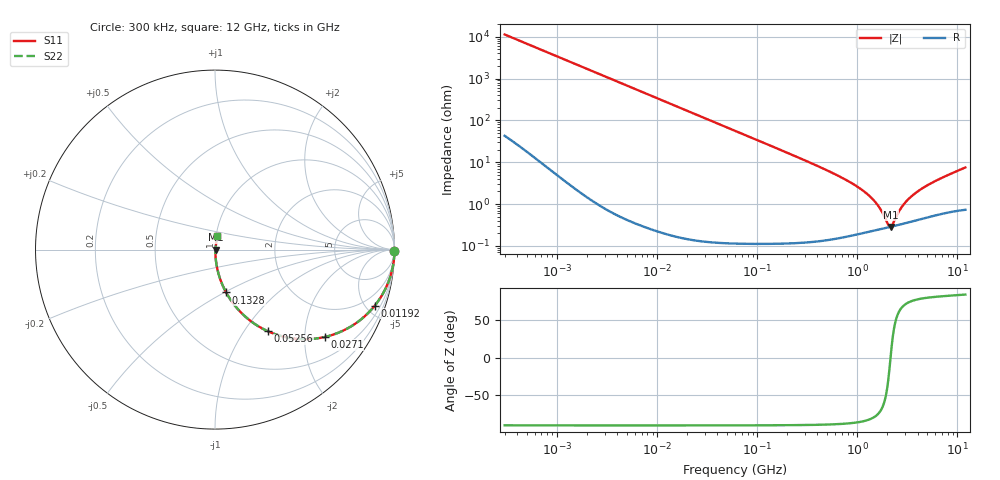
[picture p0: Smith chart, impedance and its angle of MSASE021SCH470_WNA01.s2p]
! MSASE021SCH470_WNA01  S-PARAMETER MODEL  ( Standard Model )
! Model Generated by TAIYO YUDEN Corporation (http://www.ty-top.com)
! Version 3.0
! TAIYO YUDEN Control No. 231201
! Copyright(c) 2016 TAIYO YUDEN CO.,LTD. All Rights Reserved.
! Product Description (link to TY-COMPAS)
! https://ds.yuden.co.jp/TYCOMPAS/or/detail?pn=MSASE021SCH470JWNA01&u=M
! Products Name : Multilayer Ceramic Capacitors
! Characteristics :
!  Capacitance : 47 [pF] , Rated Voltage : 16 [V] , TCC : CH / C0H
!  Case Size : 0.25 x 0.125 / 0.0098 x 0.0049 [mm/inch] , Thickness : 0.125 / 0.0049 [mm/inch]
!  (Conditions: Temperature = 25 [degC] , DC Bias Voltage = 0 [V])
! External Node Assignments :
!  1  o---| |---o  2
! GND o---------o GND
! Frequency Range : 0.3MHz  -  12000MHz  [ 401 STEP ]
# MHZ S RI R 50
! Freq[MHz].  S11 Real  S11 Imag  S21 Real  S21 Imag  S12 Real  S12 Imag  S22 Real  S22 Imag
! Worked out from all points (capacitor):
!   401 points, 300 kHz to 12 GHz, reference 50 ohm
!   read as one part in series: C = 47 pF near 316.3 kHz
!   lowest |Z| = 286 mohm at 2.145 GHz (marker M1)
!   series resonance near 2.145 GHz, so ESL is about 120 pH
!   S11 on the Smith chart (normalised r, x): 300 kHz: open; 11.92 MHz: 1.00, -5.69; 27.1 MHz: 1.00, -2.50; 52.56 MHz: 1.00, -1.29; 132.8 MHz: 1.00, -0.51; 12 GHz: 1.01, +0.15
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0.3  0.9999 -0.00886  0.000112 0.00886  0.000112 0.00886  0.9999 -0.00886
1.769972  0.9972 -0.052  0.00276 0.052  0.00276 0.052  0.9972 -0.052
4.593584  0.9819 -0.1329  0.0181 0.1329  0.0181 0.1329  0.9819 -0.1329
10.44266  0.9133 -0.281  0.0867 0.281  0.0867 0.281  0.9133 -0.281
11.92167  0.89 -0.3126  0.11 0.3126  0.11 0.3126  0.89 -0.3126
17.7384  0.7852 -0.4103  0.2148 0.4103  0.2148 0.4103  0.7852 -0.4103
27.10171  0.6104 -0.4871  0.3896 0.4871  0.3896 0.4871  0.6104 -0.4871
52.55639  0.2943 -0.4549  0.7057 0.4549  0.7057 0.4549  0.2943 -0.4549
60  0.2425 -0.4276  0.7575 0.4276  0.7575 0.4276  0.2425 -0.4276
86.94074  0.1325 -0.3376  0.8675 0.3376  0.8675 0.3376  0.1325 -0.3376
132.8329  0.0617 -0.2384  0.9383 0.2384  0.9383 0.2384  0.0617 -0.2384
353.9943  0.00977 -0.0919  0.9902 0.0919  0.9902 0.0919  0.00977 -0.0919
743.2595  0.00318 -0.0395  0.9968 0.0395  0.9968 0.0395  0.00318 -0.0395
1197.383  0.00243 -0.019  0.9976 0.019  0.9976 0.019  0.00243 -0.019
1602.47  0.00251 -0.00901  0.9975 0.00901  0.9975 0.00901  0.00251 -0.00901
2088.533  0.00281 -0.000799  0.9972 0.000799  0.9972 0.000799  0.00281 -0.000799
2144.601  0.00285 1.19e-06  0.9971 -1.19e-06  0.9971 -1.19e-06  0.00285 1.19e-06
2261.293  0.00294 0.0016  0.9971 -0.0016  0.9971 -0.0016  0.00294 0.0016
2870.14  0.00346 0.0088  0.9965 -0.0088  0.9965 -0.0088  0.00346 0.0088
3740.715  0.00427 0.0172  0.9957 -0.0172  0.9957 -0.0172  0.00427 0.0172
5868.704  0.0064 0.0337  0.9936 -0.0337  0.9936 -0.0337  0.0064 0.0337
12000  0.0127 0.0731  0.9873 -0.0731  0.9873 -0.0731  0.0127 0.0731
